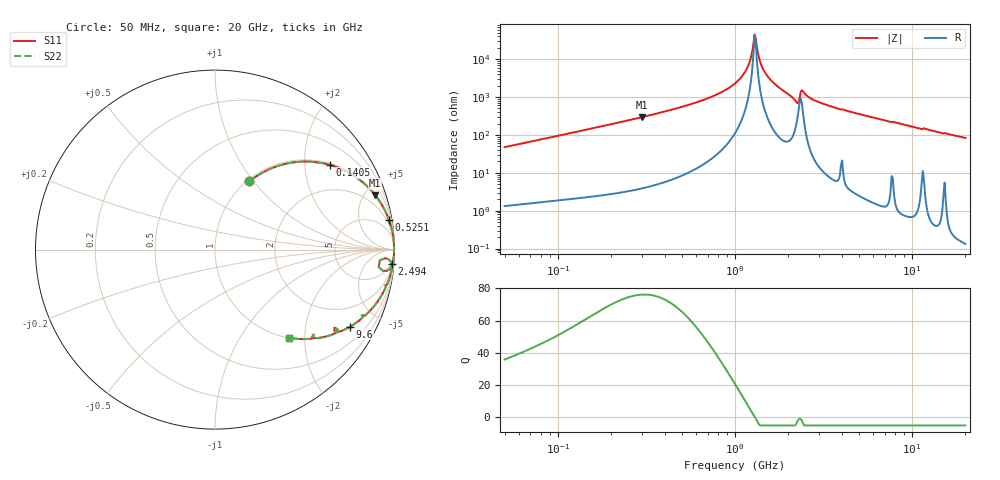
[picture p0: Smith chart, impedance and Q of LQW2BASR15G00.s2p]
!Murata Part Number: LQW2BASR15G00
!These Parameters are Measured in Series Mode Connection
!  o--[Z]--o
!Port1  Port2
!  o-------o
!Freq. Start=50[MHz] Stop=20[GHz], 401[Steps]
# Hz S RI R 50
!Freq.(Hz) S11(Real) S11(Imag) S21(Real) S21(Imag) S12(Real) S12(Imag) S22(Real) S22(Imag)
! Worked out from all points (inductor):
!   401 points, 50 MHz to 20 GHz, reference 50 ohm
!   read as one part in series: L = 151 nH near 51.52 MHz
!   highest Q = 76.1 at 297.2 MHz (marker M1), where L = 158 nH
!   self-resonance near 1.29 GHz
!   S11 on the Smith chart (normalised r, x): 50 MHz: 1.03, +0.95; 140.5 MHz: 1.04, +2.68; 525.1 MHz: 1, +12; 2.494 GHz: 4, -24; 9.6 GHz: 1.01, -3.50; 20 GHz: 1.00, -1.67
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5e7  0.1914 0.3797  0.8086 -0.3797  0.8086 -0.3797  0.1914 0.3797
1.364002e8  0.6256 0.4756  0.3744 -0.4756  0.3744 -0.4756  0.6256 0.4756
1.405482e8  0.6396 0.4719  0.3604 -0.4719  0.3604 -0.4719  0.6396 0.4719
2.972233e8  0.8933 0.3023  0.1067 -0.3023  0.1067 -0.3023  0.8933 0.3023
3.721004e8  0.9324 0.2445  0.0676 -0.2445  0.0676 -0.2445  0.9324 0.2445
5.251442e8  0.9694 0.1645  0.0306 -0.1645  0.0306 -0.1645  0.9694 0.1645
7.751977e8  0.99 0.0878  0.01 -0.0878  0.01 -0.0878  0.99 0.0878
1e9  0.996 0.0433  0.00399 -0.0433  0.00399 -0.0433  0.996 0.0433
1.161586e9  0.9976 0.0182  0.00241 -0.0182  0.00241 -0.0182  0.9976 0.0182
1.289994e9  0.9979 0.000736  0.00209 -0.000736  0.00209 -0.000736  0.9979 0.000736
1.329223e9  0.9979 -0.00429  0.00212 0.00429  0.00212 0.00429  0.9979 -0.00429
1.369645e9  0.9978 -0.00934  0.00221 0.00934  0.00221 0.00934  0.9978 -0.00934
1.432596e9  0.9976 -0.017  0.00244 0.017  0.00244 0.017  0.9976 -0.017
1.614971e9  0.9962 -0.038  0.00378 0.038  0.00378 0.038  0.9962 -0.038
2.211938e9  0.9561 -0.1183  0.0439 0.1183  0.0439 0.1183  0.9561 -0.1183
2.383959e9  0.9676 -0.0548  0.0324 0.0548  0.0324 0.0548  0.9676 -0.0548
2.493527e9  0.9837 -0.0811  0.0163 0.0811  0.0163 0.0811  0.9837 -0.0811
2.728004e9  0.9837 -0.1113  0.0163 0.1113  0.0163 0.1113  0.9837 -0.1113
3.850025e9  0.9576 -0.1947  0.0424 0.1947  0.0424 0.1947  0.9576 -0.1947
7.442007e9  0.8352 -0.3669  0.1648 0.3669  0.1648 0.3669  0.8352 -0.3669
9.600142e9  0.7534 -0.4291  0.2466 0.4291  0.2466 0.4291  0.7534 -0.4291
2e10  0.4111 -0.4912  0.5889 0.4912  0.5889 0.4912  0.4111 -0.4912
